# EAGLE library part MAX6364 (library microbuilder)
MAX6364 - Low Power Voltage Supervisor (3.08V) with Battery Backup This 'battery backup supervisor' will supply up to 150mA of current from VCC. If VCC ever drops below the 3.08V threshold, the supervisor will automatically switch the power supply to battery power, allowing you to safely 'fall-back' on a secondary power source for critical applications, or where you know that the main power suppy is inherently volatile (solar panels, etc.) Digikey: MAX6364LUT31+TCT-ND
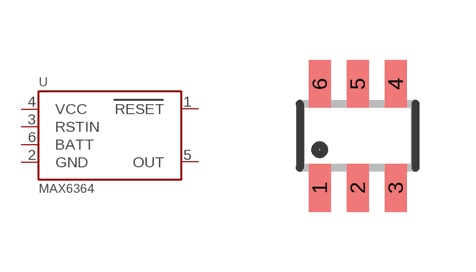
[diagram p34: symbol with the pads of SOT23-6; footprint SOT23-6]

Designator prefix U

## MAX6364  [SOT23-6]
1  RESET
2  GND  pwr
3  RSTIN
4  VCC  pwr
5  OUT
6  BATT

## Footprint SOT23-6 (pad centres in mm)
Small Outline Transistor - 6 Pin
smd 0.55 x 1.2: 1 -0.95,-1.3; 2 0,-1.3; 3 0.95,-1.3; 4 0.95,1.3; 5 0,1.3; 6 -0.95,1.3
